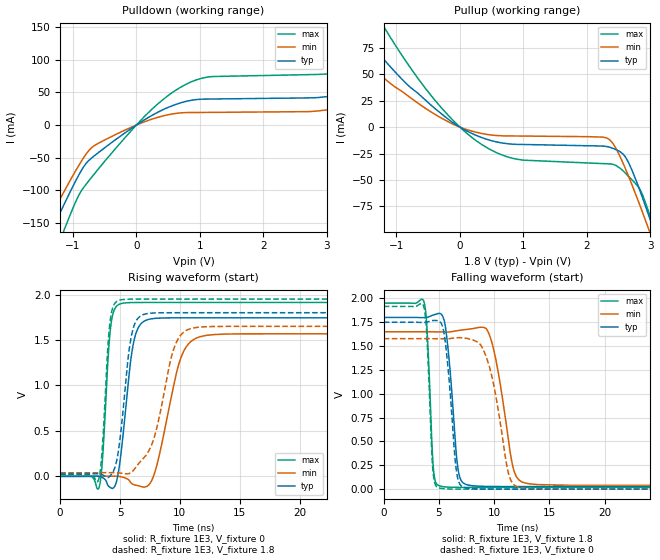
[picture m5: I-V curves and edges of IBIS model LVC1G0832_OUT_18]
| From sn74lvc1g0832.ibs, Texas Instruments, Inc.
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[Model]   LVC1G0832_OUT_18
Model_type  Output
Vref =   0
Rref =   1000
Cref =   30p
Vmeas =   0.9
| variable   typ   min   max
C_comp   9.91pF   6.37pF   16.11pF
| C_pullup   9.05pF   6.37pF   10.13pF
| C_pulldown   10.77pF   6.87pF   16.11pF
[Temperature Range]   40   100   -40
| Ambient temperature   25   85   -40
[Voltage range]   1.8   1.65   1.95
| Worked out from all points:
|   slope of the pulldown table from 0 to 0.27 V, typ, clamps not added: 16.8 ohm
|   slope of the pullup table from 0 to 0.27 V, typ, clamps not added: 33 ohm
|   rising waveform, R_fixture 1E3, V_fixture 0: 20-80 % time 861ps typ, 1.54ns min, 499ps max; typ from 0 V to 1.74 V
|   falling waveform, R_fixture 1E3, V_fixture 1.8: 20-80 % time 715ps typ, 1.29ns min, 423ps max; typ from 1.8 V to 0.027 V
|   rising waveform, R_fixture 1E3, V_fixture 1.8: 20-80 % time 851ps typ, 1.64ns min, 497ps max; typ from 0.027 V to 1.8 V
|   falling waveform, R_fixture 1E3, V_fixture 0: 20-80 % time 722ps typ, 1.42ns min, 417ps max; typ from 1.75 V to 0 V
[Pulldown]
| LVC1G0832_OUT_18
|   Voltage   I(typ)   I(min)   I(max)
-5.5V     -1.02A     -914.2mA   -1.211A
-1.49V    -194.3mA   -166.1mA   -248.7mA
-1.27V    -148.7mA   -125.7mA   -193.7mA
-1.11V    -116mA     -96.9mA    -154.1mA
-645mV    -45.9mA    -30.54mA   -72.92mA
690mV     33.84mA    18.58mA    57.6mA
1.17V     39.88mA    19.4mA     74.12mA
3.205V    47.28mA    26.68mA    81.73mA
4.215V    77.94mA    21.52mA    128.8mA
4.595V    44.42mA    21.74mA    150.4mA
5.01V     44.71mA    21.98mA    83.24mA
11V       50.71mA    25.31mA    93.17mA
[Pullup]
| LVC1G0832_OUT_18
|   Voltage   I(typ)   I(min)   I(max)
-5.5V     449.7mA    254mA      638.5mA
-2.225V   143.3mA    107.6mA    207.3mA
-1.755V   105.1mA    78.04mA    153.5mA
-1.195V   63.95mA    46.44mA    94.81mA
-375mV    16.75mA    11.48mA    24.15mA
420mV     -11.47mA   -6.842mA   -19.31mA
2.34V     -18.75mA   -11.19mA   -34.79mA
2.61V     -28.71mA   -39.94mA   -43.87mA
2.825V    -58.63mA   -72.76mA   -58mA
2.97V     -83.15mA   -96.31mA   -80.03mA
3.12V     -109.8mA   -121.4mA   -108.9mA
11V       -1.703A    -1.583A    -1.935A
[Ramp]
| LVC1G0832_OUT_18
| variable   typ   min   max
dV/dt_r   1.13/9.23E-10   1.01/1.65E-09   1.23/5.40E-10
dV/dt_f   1.09/7.41E-10   1.00/1.34E-09   1.18/4.40E-10
R_load = 1E3
[Rising Waveform]
| LVC1G0832_OUT_18
R_fixture =   1E3
C_fixture =   0
L_fixture =   0
V_fixture =   0
V_fixture_min = 0
V_fixture_max = 0
|   Time   V(typ)   V(min)   V(max)
0s        114pV      8.171nV    2.621nV
3.25ns    1.297mV    19.31uV    -122.4mV
3.53ns    -12.46mV   764.7uV    178.6mV
4.215ns   -125mV     1.388mV    1.639V
5.085ns   252.8mV    -4.986mV   1.9V
6.13ns    1.469V     -90.49mV   1.912V
7.4ns     1.727V     -95.14mV   1.913V
10.04ns   1.744V     1.286V     1.913V
11.69ns   1.744V     1.536V     1.913V
50ns      1.744V     1.568V     1.913V
[Falling Waveform]
| LVC1G0832_OUT_18
R_fixture =   1E3
C_fixture =   0
L_fixture =   0
V_fixture =   1.8
V_fixture_min = 1.65
V_fixture_max = 1.95
|   Time   V(typ)   V(min)   V(max)
0s        1.8V       1.65V      1.95V
3.645ns   1.798V     1.65V      1.965V
4.49ns    1.825V     1.649V     231.6mV
5.015ns   1.843V     1.648V     36.41mV
5.7ns     1.603V     1.647V     22.37mV
6.73ns    212.7mV    1.663V     18.84mV
7.435ns   49.87mV    1.673V     18.42mV
9.58ns    28.66mV    1.615V     18.24mV
12.69ns   27.37mV    68.3mV     18.23mV
50ns      27.29mV    39.56mV    18.21mV
[Rising Waveform]
| LVC1G0832_OUT_18
R_fixture =   1E3
C_fixture =   0
L_fixture =   0
V_fixture =   1.8
V_fixture_min = 1.65
V_fixture_max = 1.95
|   Time   V(typ)   V(min)   V(max)
0s        27.26mV    39.51mV    18.19mV
3.195ns   28.79mV    39.48mV    -41.18mV
4.16ns    3.968mV    40.65mV    1.691V
4.965ns   374.2mV    37.22mV    1.938V
5.775ns   1.401V     31.35mV    1.949V
6.35ns    1.71V      105.2mV    1.95V
7.805ns   1.797V     407mV      1.95V
9.605ns   1.8V       1.443V     1.95V
10.94ns   1.8V       1.626V     1.95V
50ns      1.8V       1.65V      1.95V
[Falling Waveform]
| LVC1G0832_OUT_18
R_fixture =   1E3
C_fixture =   0
L_fixture =   0
V_fixture =   0
V_fixture_min = 0
V_fixture_max = 0
|   Time   V(typ)   V(min)   V(max)
0s        1.749V     1.578V     1.916V
3.63ns    1.748V     1.578V     1.913V
4.45ns    1.768V     1.577V     205.9mV
4.97ns    1.764V     1.577V     14.7mV
5.61ns    1.511V     1.577V     3.483mV
6.605ns   174.7mV    1.587V     518.7uV
7.275ns   17.78mV    1.585V     186.4uV
9.285ns   940uV      1.386V     46.11uV
12.18ns   86.68uV    20.94mV    36.61uV
50ns      22.27uV    42.4uV     11.55uV
